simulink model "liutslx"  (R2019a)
settings: configuration reference "configurationSettings" (kept in a data dictionary, not in this file)
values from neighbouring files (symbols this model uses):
  ag = NaN(L.ng,1)    [bdet.m]
  D = meqp()    [fbtp.m]
  dr2FA = dr2Fs(1:nA,1)    [asxycs.m]
  drzFA = drzFs(1:nA,1)    [asxycs.m]
  dz = dzxs(is)    [asxycsJac.m]    (also in bintc.m = (z - zx(kz))/dzx)
  dz2FA = dz2Fs(1:nA,1)    [asxycs.m]
  err = [IaeH            ; IoeH               ; IueH               ; DeH               ; FeH            ; BeH               ; BeH               ; BeH               ; CeH               ; CeH               ; CeH               ; VeH                ; VeH                ; VeH               ]    [fbtopt.m]
  FA = Fs(1:nA,1)    [asxycs.m]    (also in bfhelp.m = [-1                        0        0       ])
  FB = [0                         1        1       ]    [bfhelp.m]
  Fx = meqFx(L,Iy,[Ia;Iu])    [bdet.m]    (also in bfhelp.m = zeros(n+2,3); Fx(2:end-1,2) = FN)
  FX = Fs(nA+1:ns,1)    [asxycs.m]
  Iy = LXt.Iy    [bdet.m]    (also in fbtinit.m = meqinitIy(L,LXs.t,IpD,bbs,LXs.capaj))
  L = fbtc(P,G)    [fbt.m]    (also in fbtc.m = meqc(P,G); fbte.m = varargout{1})
  nA = numel(rA)    [asxycs.m]
  niter = L.P.itercs    [asxycs.m]
  Opy = logical(Opy)    [bfct.m]    (also in bfdoublet.m = Opy==1 | Opy==2)
  rA = rs(1:nA,1)    [asxycs.m]    (also in fbtptcv.m = (rA1 + 3*rA2)/4)
  rX = rs(nA+1:ns,1)    [asxycs.m]    (also in fbtptcv.m = rzbro(iX,1); fbtxana.m = r0)
  zA = zs(1:nA,1)    [asxycs.m]    (also in fbtptcv.m = (zA1 + 3*zA2)/4)
  zX = zs(nA+1:ns,1)    [asxycs.m]    (also in fbtptcv.m = rzbro(iX,2); fbtxana.m = 0)
undefined symbols (not defined in the file or in its folder): Bm, bp, bpli2, Brn, Brrn, Brzn, bt, Bzn, Bzrn, Bzzn, dzg, Ff, Fn, Ft, Ft0, Ie, Ip, iTQ, lB, li, lX, mu, nX, PpQ, PQ, rB, rBt, repmat, Row, rst, TQ, TTpQ, Un, vector, Vp, Wk, WN, Wp, Wt, Wt0, zB
libraries: liulib x34, mkllib x28, simulink x5
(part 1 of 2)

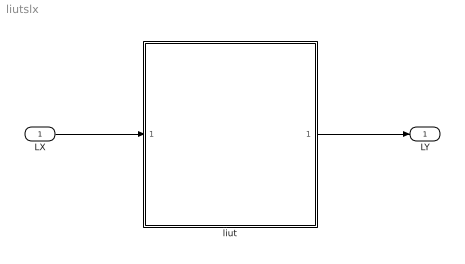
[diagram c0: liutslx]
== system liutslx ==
  LX : Inport  OutDataTypeStr=Bus: LXbus  PortDimensions=1  SampleTime=L.dt  Interpolate=off
  liut : Subsystem  AncestorBlock=liulib/liut  TreatAsAtomicUnit=on
  LY : Outport  OutDataTypeStr=Bus: LYbus  PortDimensions=1
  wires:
  LX/1 -> liut/1(LX)
  liut/1(LY) -> LY/1

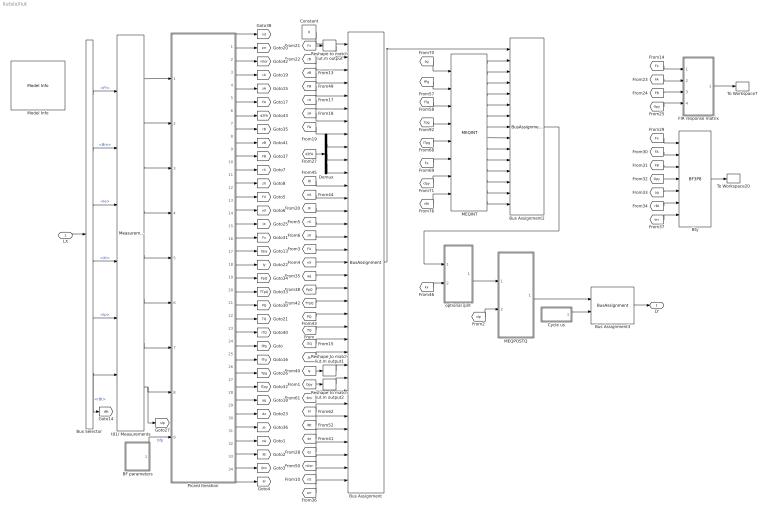
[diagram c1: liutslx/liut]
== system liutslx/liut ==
  LX : Inport
  BF parameters : Subsystem  Variant=on  VariantControl=Variant1
  Bty : liulib/BF3P8  Commented=on  ids=L.idsx  iry=L.iry
  Bus Assignment : BusAssignment  AssignedSignals=Fx,rB,zB,FB,rA,zA,FA,dr2FA,dz2FA,drzFA,lB,nA,lX,rX,zX,FX,nX,ag,PpQ,TTpQ,PQ,TQ,iTQ,Ie,Iy,Opy,Bm,Ff,rBt,dz,dzg,niter,rst,err
  Bus Assignment2 : BusAssignment  AssignedSignals=Ip,Wk,Wp,Wt,Wt0,Ft,Ft0,Vp,bp,bt,mu,li,bpli2,WN
  Bus Assignment3 : BusAssignment  AssignedSignals=cycle
  Bus Selector : BusSelector  OutputSignals=Ff,Bm,Ie,Xt,Ip,rBt
  Constant : Constant  Value=0  OutDataTypeStr=Bus: LYbus
  Cycle us : Subsystem
  Demux : Demux  Outputs=3
  FIR response matrix : Subsystem  Commented=on
  MEQINT : liulib/MEQINT  SystemSampleTime=-1
  MEQPOSTQ : Subsystem  Variant=on  VariantControl=Variant1
  Model Info : simulink/Model-Wide Utilities/Model Info  Frame=on  DisplayStringWithTags=|  HorizontalTextAlignment=Center  LeftAlignmentValue=0.5
      | Model Info
      | %<Creator>
      | %<ModifiedBy>
      | %<ModifiedDate>
      | %<ModifiedComment>
      | %<ModelVersion>
  Picard Iteration : Subsystem
  Reshape to match liut.m output : Reshape  OutputDimensionality=Customize  OutputDimensions=[L.nzx,L.nrx]
  Reshape to match liut.m output1 : Reshape  OutputDimensionality=Customize  OutputDimensions=[L.nzy,L.nry]
  Reshape to match liut.m output2 : Reshape  OutputDimensionality=Customize  OutputDimensions=[L.nzy,L.nry]
  To Workspace20 : ToWorkspace  VariableName=Bty  SampleTime=-1
  To Workspace7 : ToWorkspace  VariableName=Tdg  SampleTime=-1
  optional qint : Subsystem  Variant=on  VariantControl=Variant1
  t01/ Measurements : liulib/t01// Measurements  SystemSampleTime=-1
  LY : Outport
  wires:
  Picard Iteration/13(Out31) -> [FX]
  t01/ Measurements/5 -> Picard Iteration/5(Ip)
  Reshape to match liut.m output2/1 -> Bus Assignment/27
  [Opy] -> Reshape to match liut.m output2/1
  [err] -> Bus Assignment/35
  [rst] -> Bus Assignment/34
  [niter] -> Bus Assignment/33
  [dz] -> Bus Assignment/32
  [dz] -> Bus Assignment/31
  [Ff] -> Bus Assignment/29
  [rBt] -> Bus Assignment/30
  [Bm] -> Bus Assignment/28
  MEQPOSTQ/1(" LYo") -> Bus Assignment3/1
  [sIp] -> MEQPOSTQ/2("sIp ")
  optional qint/1(" LYo") -> MEQPOSTQ/1("LY ")
  t01/ Measurements/1 -> Picard Iteration/1(Yr)
  Bus Selector/2 -> t01/ Measurements/2  "<Bm>"
  Bus Selector/1 -> t01/ Measurements/1  "<Ff>"
  t01/ Measurements/2 -> Picard Iteration/2(Yd)
  t01/ Measurements/3 -> Picard Iteration/3(Yi)
  t01/ Measurements/6 -> Picard Iteration/6(rBt)
  t01/ Measurements/7 -> Picard Iteration/7(FN)
  t01/ Measurements/8 -> [sIp], Picard Iteration/8(sIp)
  BF parameters/1(" bfp") -> Picard Iteration/9(bfp)  "bfp"
  LX/1 -> Bus Selector/1
  Bus Selector/5 -> t01/ Measurements/5  "<Ip>"
  Bus Selector/3 -> t01/ Measurements/3  "<Ie>"
  t01/ Measurements/4 -> Picard Iteration/4(Ie)
  MEQINT/5 -> Bus Assignment2/6
  [ag] -> MEQINT/1
  [Opy] -> MEQINT/7
  [fTg] -> MEQINT/3
  MEQINT/3 -> Bus Assignment2/4
  [fPg] -> MEQINT/2
  MEQINT/6 -> Bus Assignment2/7
  [rBt] -> MEQINT/8
  MEQINT/9 -> Bus Assignment2/10
  MEQINT/7 -> Bus Assignment2/8
  MEQINT/12 -> Bus Assignment2/13
  MEQINT/1 -> Bus Assignment2/2
  [Fx] -> MEQINT/6
  MEQINT/2 -> Bus Assignment2/3
  [Tpg] -> MEQINT/4
  MEQINT/4 -> Bus Assignment2/5
  [ITpg] -> MEQINT/5
  MEQINT/8 -> Bus Assignment2/9
  MEQINT/11 -> Bus Assignment2/12
  MEQINT/10 -> Bus Assignment2/11
  Constant/1 -> Bus Assignment/1
  Picard Iteration/8(Out9) -> [rB]
  Picard Iteration/6(Out7) -> [FA]
  Picard Iteration/24(Out19) -> [fPg]
  Picard Iteration/9(Out10) -> [zB]
  Picard Iteration/4(Out5) -> [rA]
  Picard Iteration/2(Out2) -> [err]
  Picard Iteration/21(Out16) -> [PQ]
  Picard Iteration/7(Out8) -> [d2FA]
  Picard Iteration/25(Out20) -> [fTg]
  Picard Iteration/26(Out21) -> [Tpg]
  Picard Iteration/28(Out23) -> [ag]
  Picard Iteration/16(Out13) -> [Fx]
  Picard Iteration/3(Out3) -> [niter]
  Picard Iteration/1(Out1) -> [rst]
  Picard Iteration/15(Out12) -> [lX]
  Picard Iteration/17(Out14) -> [Opy]
  Picard Iteration/22(Out17) -> [TQ]
  Picard Iteration/27(Out22) -> [ITpg]
  Picard Iteration/10(Out11) -> [FB]
  Picard Iteration/20(Out26) -> [TTpQ]
  Picard Iteration/30(Out4) -> [Je]
  Picard Iteration/5(Out6) -> [zA]
  Picard Iteration/18(Out15) -> [Iy]
  Picard Iteration/29(Out24) -> [dz]
  Picard Iteration/19(Out25) -> [PpQ]
  Picard Iteration/23(Out18) -> [iTQ]
  [rA] -> Bus Assignment/6
  [zA] -> Bus Assignment/7
  [FA] -> Bus Assignment/8
  Demux/1 -> Bus Assignment/9
  Demux/3 -> Bus Assignment/11
  Demux/2 -> Bus Assignment/10
  [d2FA] -> Demux/1
  [FB] -> Bus Assignment/5
  [zB] -> Bus Assignment/4
  [rB] -> Bus Assignment/3
  [Fx] -> Reshape to match liut.m output/1
  Picard Iteration/31(Out27) -> [nA]
  Picard Iteration/32(Out28) -> [lB]
  [lB] -> Bus Assignment/12
  [nA] -> Bus Assignment/13
  [ag] -> Bus Assignment/19
  [lX] -> Bus Assignment/14
  [PpQ] -> Bus Assignment/20
  [TTpQ] -> Bus Assignment/21
  [PQ] -> Bus Assignment/22
  [TQ] -> Bus Assignment/23
  Bus Assignment/1 -> Bus Assignment2/1
  MEQINT/13 -> Bus Assignment2/14
  Reshape to match liut.m output/1 -> Bus Assignment/2
  Cycle us/1(Out1) -> Bus Assignment3/2
  Bus Assignment3/1 -> LY/1
  [err] -> Bty/7
  [FB] -> Bty/3
  [Fx] -> Bty/1
  [FB] -> FIR response matrix/3(FB)
  [ag] -> Bty/5
  [Fx] -> FIR response matrix/1(Fx)
  Bty/1 -> To Workspace20/1
  [rBt] -> Bty/6
  [Opy] -> Bty/4
  FIR response matrix/1(Tdg) -> To Workspace7/1
  [FA] -> FIR response matrix/2(FA)
  [FA] -> Bty/2
  [Opy] -> FIR response matrix/4(Opy)
  Bus Selector/4 -> t01/ Measurements/4  "<Xt>"
  Bus Selector/6 -> [rBt], t01/ Measurements/6  "<rBt>"
  [Je] -> Bus Assignment/25
  [Iy] -> Reshape to match liut.m output1/1
  Reshape to match liut.m output1/1 -> Bus Assignment/26
  [iTQ] -> Bus Assignment/24
  MEQINT/14 -> Bus Assignment2/15
  Picard Iteration/33(Out29) -> [Bm]
  Picard Iteration/34(Out30) -> [Ff]
  [Fx] -> optional qint/2(Fx)
  Bus Assignment2/1 -> optional qint/1("LY ")
  [FX] -> Bus Assignment/17
  Picard Iteration/14(Out32) -> [nX]
  [nX] -> Bus Assignment/18
  Picard Iteration/11(Out33) -> [rX]
  Picard Iteration/12(Out34) -> [zX]
  [rX] -> Bus Assignment/15
  [zX] -> Bus Assignment/16

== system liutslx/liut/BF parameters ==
  BF3I : Subsystem  VariantControl=liuBFCTMODEvariant2
  BF3P : Subsystem  VariantControl=liuBFCTMODEvariant1
  BFEF : Subsystem  VariantControl=liuBFCTMODEvariant3
  " bfp" : Outport

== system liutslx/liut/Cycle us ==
  Data Type Conversion : DataTypeConversion
  Memory : Memory  InheritSampleTime=on
  Sum : Sum  Inputs=|+-
  Wall time : liulib/Wall time  f=1000000
  Out1 : Outport  OutDataTypeStr=single
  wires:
  Wall time/1 -> Sum/1, Memory/1
  Sum/1 -> Data Type Conversion/1
  Memory/1 -> Wall time/1, Sum/2
  Data Type Conversion/1 -> Out1/1

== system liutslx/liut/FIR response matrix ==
  Fx : Inport
  FA : Inport  Port=2
  FB : Inport  Port=3
  Opy : Inport  Port=4
  BF3I4 : liulib/BF3I4  nzy=L.nzy  nry=L.nry
  Constant : Constant  Value=ones(21,3)  VectorParams1D=off  OutDataTypeStr=single
  Constant1 : Constant  Value=0:9  OutDataTypeStr=uint32
  Constant2 : Constant  Value=[ones(10,1) zeros(10,1)]  OutDataTypeStr=single
  Terminator : Terminator
  Tdg : Outport
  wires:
  BF3I4/2 -> Terminator/1
  Fx/1 -> BF3I4/1
  Opy/1 -> BF3I4/4
  Constant2/1 -> BF3I4/7
  FA/1 -> BF3I4/2
  Constant1/1 -> BF3I4/6
  Constant/1 -> BF3I4/5
  BF3I4/1 -> Tdg/1
  FB/1 -> BF3I4/3

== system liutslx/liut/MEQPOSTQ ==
  "LY " : Inport
  "sIp " : Inport  Port=2
  Direct pass : Subsystem  VariantControl=liuITERQMODEvariant0
  MEQPOSTQ : liulib/MEQPOSTQ  SystemSampleTime=-1  VariantControl=liuITERQMODEvariant1
  " LYo" : Outport

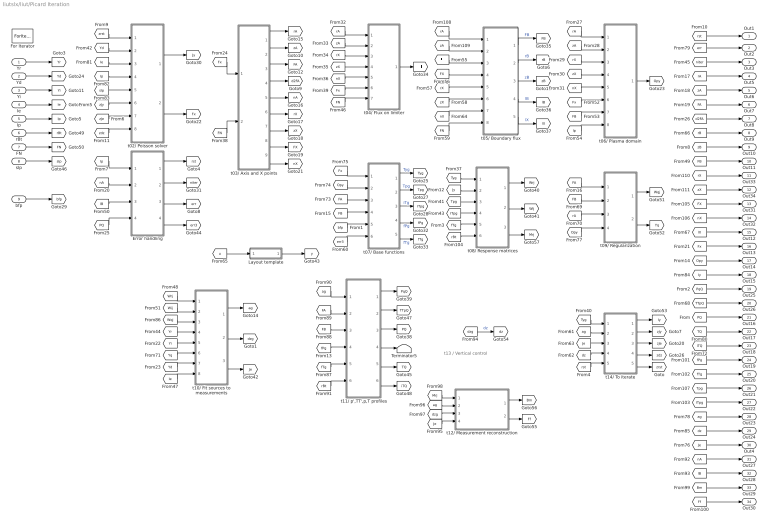
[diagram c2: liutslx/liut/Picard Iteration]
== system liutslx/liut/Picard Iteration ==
  note: t13 / Vertical control
  Yr : Inport
  Yd : Inport  Port=2
  Yi : Inport  Port=3
  Ie : Inport  Port=4
  Ip : Inport  Port=5
  rBt : Inport  Port=6
  FN : Inport  Port=7
  sIp : Inport  Port=8
  bfp : Inport  Port=9
  Error handling : Subsystem
  For Iterator : ForIterator  IterationLimit=L.P.itert  ShowIterationPort=off
  Layout template : Subsystem  Commented=on
  Terminator5 : Terminator
  t02/ Poisson solver : Subsystem
  t03/ Axis and X points : Subsystem  TreatAsAtomicUnit=on
  t04/ Flux on limiter : Subsystem
  t05/ Boundary flux : Subsystem
  t06/ Plasma domain : Subsystem
  t07/ Base functions : Subsystem  Variant=on
  t08/ Response matrices : Subsystem
  t09/ Regularization : Subsystem  TreatAsAtomicUnit=on
  t10/ Fit sources to measurements : Subsystem  Variant=on  VariantControl=Variant1
  t11/ p',TT',p,T profiles : Subsystem  VariantControl=Variant1
  t12/ Measurement reconstruction : Subsystem
  t14/ To iterate : Subsystem
  Out1 : Outport
  Out2 : Outport  Port=2
  Out3 : Outport  Port=3
  Out5 : Outport  Port=4
  Out6 : Outport  Port=5
  Out7 : Outport  Port=6
  Out8 : Outport  Port=7
  Out9 : Outport  Port=8
  Out10 : Outport  Port=9
  Out11 : Outport  Port=10
  Out33 : Outport  Port=11
  Out34 : Outport  Port=12
  Out31 : Outport  Port=13
  Out32 : Outport  Port=14
  Out12 : Outport  Port=15
  Out13 : Outport  Port=16
  Out14 : Outport  Port=17
  Out15 : Outport  Port=18
  Out25 : Outport  Port=19
  Out26 : Outport  Port=20
  Out16 : Outport  Port=21
  Out17 : Outport  Port=22
  Out18 : Outport  Port=23
  Out19 : Outport  Port=24
  Out20 : Outport  Port=25
  Out21 : Outport  Port=26
  Out22 : Outport  Port=27
  Out23 : Outport  Port=28
  Out24 : Outport  Port=29
  Out4 : Outport  Port=30
  Out27 : Outport  Port=31
  Out28 : Outport  Port=32
  Out29 : Outport  Port=33
  Out30 : Outport  Port=34
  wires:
  [rA] -> t05/ Boundary flux/1(rA)
  [zA] -> t05/ Boundary flux/2(zA)
  t05/ Boundary flux/5(lX) -> [lX]  "lX"
  t05/ Boundary flux/1(FB) -> [FB]  "FB"
  t05/ Boundary flux/4(lB) -> [lB]  "lB"
  t05/ Boundary flux/3(zB) -> [zB]  "zB"
  t05/ Boundary flux/2(rB) -> [rB]  "rB"
  [FN] -> t05/ Boundary flux/8(FN)
  [zX] -> t05/ Boundary flux/6(zX)
  [rX] -> t05/ Boundary flux/5(rX)
  [Fl] -> t05/ Boundary flux/3(Fl)
  [FX] -> t05/ Boundary flux/4(FX)
  [nX] -> t05/ Boundary flux/7(nX)
  [FX] -> Out31/1
  [rBt] -> t08/ Response matrices/6(rBt)
  [Je] -> Out4/1
  [Wqj] -> t10/ Fit sources to measurements/3(Wqj)
  [Yq] -> t10/ Fit sources to measurements/6(Yq)
  [FA] -> t09/ Regularization/1(FA)
  [FB] -> t09/ Regularization/2(FB)
  [Opy] -> t09/ Regularization/4(Opy)
  [rA] -> t09/ Regularization/3(rA)
  t09/ Regularization/2(Yq) -> [Yq]
  t09/ Regularization/1(Wqj) -> [Wqj]
  t10/ Fit sources to measurements/3(Je) -> [Je]
  t10/ Fit sources to measurements/2(dzg) -> [dzg]
  t10/ Fit sources to measurements/1(ag) -> [ag]
  [Ie] -> t10/ Fit sources to measurements/8(Ie)
  [Yd] -> t10/ Fit sources to measurements/7(Yd)
  [Yi] -> t10/ Fit sources to measurements/5(Yi)
  [Yr] -> t10/ Fit sources to measurements/4(Yr)
  [Wij] -> t10/ Fit sources to measurements/2(Wij)
  [Wrj] -> t10/ Fit sources to measurements/1(Wrj)
  Error handling/4(err3) -> [err3]
  t07/ Base functions/3(ITpg) -> [ITpg]  "iTg"
  t07/ Base functions/2(Tpg) -> [Tpg]  "Tpg"
  [zA] -> t04/ Flux on limiter/2(zA)
  [rA] -> t04/ Flux on limiter/1(rA)
  [u] -> Layout template/1(u)
  Layout template/1(y) -> [y]
  [PQ] -> Out16/1
  [Iy] -> Out15/1
  [PQ] -> Error handling/4(PQ)
  [nA] -> Error handling/2(nA)
  [Ip] -> Error handling/1(Ip)
  [Fx] -> Out13/1
  [FB] -> Out11/1
  [Opy] -> Out14/1
  t11/ p',TT',p,T profiles/3(PQ) -> [PQ]
  [lX] -> Out12/1
  [rB] -> Out9/1
  [rA] -> Out5/1
  [zA] -> Out6/1
  t04/ Flux on limiter/1(Fl) -> [Fl]
  [ITpg] -> t08/ Response matrices/4(ITpg)
  [fPg] -> Out19/1
  [fTg] -> Out20/1
  [Tpg] -> Out21/1
  [nX] -> t04/ Flux on limiter/5(nX)
  [rX] -> t04/ Flux on limiter/3(rX)
  [zX] -> t04/ Flux on limiter/4(zX)
  [rX] -> t06/ Plasma domain/3(rX)
  [rA] -> t06/ Plasma domain/1(rA)
  [fTg] -> t11/ p',TT',p,T profiles/5(fTg)
  [FB] -> t11/ p',TT',p,T profiles/3(FB)
  [zrst] -> t02/ Poisson solver/1(rst)
  Ie/1 -> [Ie]
  Yd/1 -> [Yd]
  [Fx] -> t04/ Flux on limiter/6(Fx)
  [FN] -> t04/ Flux on limiter/7(FN)
  bfp/1 -> [bfp]
  Ip/1 -> [Ip]
  Yi/1 -> [Yi]
  Yr/1 -> [Yr]
  [zJe] -> t02/ Poisson solver/7(zJe)
  [Yd] -> t02/ Poisson solver/2(Yd)
  [zJy] -> t02/ Poisson solver/6(zJy)
  [iTQ] -> Out18/1
  t11/ p',TT',p,T profiles/6(iTQ) -> [iTQ]
  t11/ p',TT',p,T profiles/5(TQ) -> [TQ]
  [nX] -> t06/ Plasma domain/5(nX)
  [zX] -> t06/ Plasma domain/4(zX)
  [zA] -> t06/ Plasma domain/2(zA)
  t08/ Response matrices/2(Wij) -> [Wij]
  [fTg] -> t08/ Response matrices/5(fTg)
  t11/ p',TT',p,T profiles/4(hqTQ) -> Terminator5/1
  t11/ p',TT',p,T profiles/2(TTpQ) -> [TTpQ]
  t11/ p',TT',p,T profiles/1(PpQ) -> [PqQ]
  [Tpg] -> t08/ Response matrices/3(Tpg)
  [Tyg] -> t08/ Response matrices/1(Tyg)
  t06/ Plasma domain/1(Opy) -> [Opy]
  [Jy] -> t08/ Response matrices/2(Jy)
  [rst] -> Out1/1
  [sIp] -> t02/ Poisson solver/5(sIp)
  sIp/1 -> [sIp]
  t07/ Base functions/5(fTg) -> [fTg]  "fTg"
  t07/ Base functions/4(fPg) -> [fPg]  "fPg"
  [bfp] -> t07/ Base functions/5(bfp)
  t07/ Base functions/1(Tyg) -> [Tyg]  "Tyg"
  [err3] -> t07/ Base functions/6(err)
  [FB] -> t07/ Base functions/4(FB)
  [FA] -> Out7/1
  [d2FA] -> Out8/1
  [ag] -> Out23/1
  [err] -> Out2/1
  [rBt] -> t11/ p',TT',p,T profiles/6(rBt)
  [Ip] -> t02/ Poisson solver/4(Ip)
  [Ie] -> t02/ Poisson solver/3(Ie)
  [TQ] -> Out17/1
  [Ip] -> t06/ Plasma domain/8(Ip)
  [FB] -> t06/ Plasma domain/7(FB)
  [Fx] -> t06/ Plasma domain/6(Fx)
  Error handling/3(err) -> [err]
  [lB] -> Error handling/3(lB)
  [niter] -> Out3/1
  [dz] -> Out24/1
  t02/ Poisson solver/2(Fx) -> [Fx]
  [zdz] -> t02/ Poisson solver/8(zdz)
  t02/ Poisson solver/1(Jy) -> [Jy]
  [FA] -> t07/ Base functions/3(FA)
  [Opy] -> t07/ Base functions/2(Opy)
  [Fx] -> t07/ Base functions/1(Fx)
  t08/ Response matrices/1(Wrj) -> [Wrj]
  Error handling/1(rst) -> [rst]
  Error handling/2(niter) -> [niter]
  [zB] -> Out10/1
  FN/1 -> [FN]
  rBt/1 -> [rBt]
  [ITpg] -> Out22/1
  [FA] -> t11/ p',TT',p,T profiles/2(FA)
  [ag] -> t11/ p',TT',p,T profiles/1(ag)
  [fPg] -> t11/ p',TT',p,T profiles/4(fPg)
  [rst] -> t14/ To iterate/5(rst)
  [ag] -> t14/ To iterate/2(ag)
  [Tyg] -> t14/ To iterate/1(Tyg)
  [Je] -> t14/ To iterate/3(Je)
  [dz] -> t14/ To iterate/4(dz)
  t14/ To iterate/2(zJy) -> [zJy]
  t14/ To iterate/3(zJe) -> [zJe]
  t14/ To iterate/4(zdz) -> [zdz]
  t14/ To iterate/5(zrst) -> [zrst]
  [PqQ] -> Out25/1
  [TTpQ] -> Out26/1
  t14/ To iterate/1(Iy) -> [Iy]
  [nA] -> Out27/1
  [lB] -> Out28/1
  [dzg] -> [dz]  "dz"
  t12/ Measurement reconstruction/1(Bm) -> [Bm]
  t12/ Measurement reconstruction/2(Ff) -> [Ff]
  [Mrj] -> t12/ Measurement reconstruction/1(Mrj)
  [ag] -> t12/ Measurement reconstruction/2(ag)
  [dzg] -> t12/ Measurement reconstruction/3(dzg)
  t08/ Response matrices/3(Mrj) -> [Mrj]
  [Je] -> t12/ Measurement reconstruction/4(Ie)
  [Ff] -> Out30/1
  [Bm] -> Out29/1
  [nX] -> Out32/1
  [rX] -> Out33/1
  [zX] -> Out34/1
  [Fx] -> t03/ Axis and X points/1(Fx)
  [FN] -> t03/ Axis and X points/2(FN)
  t03/ Axis and X points/1(rA) -> [rA]
  t03/ Axis and X points/2(zA) -> [zA]
  t03/ Axis and X points/3(FA) -> [FA]
  t03/ Axis and X points/4(d2FA) -> [d2FA]
  t03/ Axis and X points/5(nA) -> [nA]
  t03/ Axis and X points/6(rX) -> [rX]
  t03/ Axis and X points/7(zX) -> [zX]
  t03/ Axis and X points/8(FX) -> [FX]
  t03/ Axis and X points/9(nX) -> [nX]

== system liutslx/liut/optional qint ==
  "LY " : Inport
  Fx : Inport  Port=2
  direct pass : Subsystem  VariantControl=liuINFCTMODEvariant1
  "qint " : Subsystem  VariantControl=liuINFCTMODEvariant2
  " LYo" : Outport

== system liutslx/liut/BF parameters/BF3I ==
  BF3I parameters : Subsystem
  Bus Creator : BusCreator  Inputs=4
  bfp : Outport
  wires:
  BF3I parameters/1(gNg) -> Bus Creator/1
  Bus Creator/1 -> bfp/1
  BF3I parameters/3(fPg) -> Bus Creator/3
  BF3I parameters/4(fTg) -> Bus Creator/4
  BF3I parameters/2(IgNg) -> Bus Creator/2

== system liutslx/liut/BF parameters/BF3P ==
  Constant : Constant  Value=L.P.bfp
  bfp : Outport
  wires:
  Constant/1 -> bfp/1

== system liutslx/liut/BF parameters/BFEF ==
  Constant : Constant  Value=L.P.bfp
  bfp : Outport
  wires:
  Constant/1 -> bfp/1

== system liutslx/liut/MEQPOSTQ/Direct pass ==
  "LY " : Inport
  "sIp " : Inport  Port=2
  Terminator : Terminator
  " LYo" : Outport
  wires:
  "sIp "/1 -> Terminator/1
  "LY "/1 -> " LYo"/1

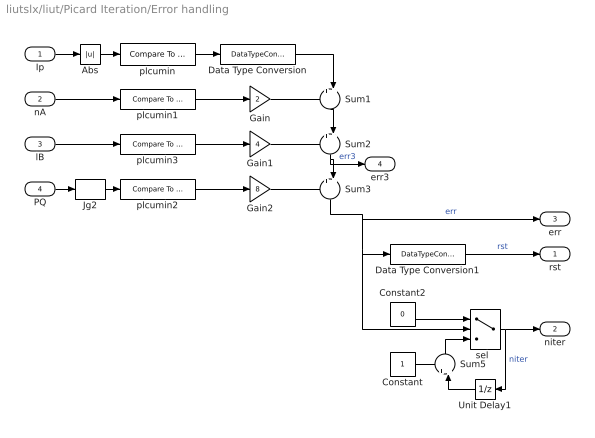
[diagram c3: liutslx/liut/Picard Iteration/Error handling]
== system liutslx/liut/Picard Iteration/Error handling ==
  Ip : Inport
  nA : Inport  Port=2
  lB : Inport  Port=3
  PQ : Inport  Port=4
  Abs : Abs
  Constant : Constant  VectorParams1D=off  OutDataTypeStr=int32
  Constant2 : Constant  Value=0  VectorParams1D=off  OutDataTypeStr=int32
  Data Type Conversion : DataTypeConversion  OutDataTypeStr=int32
  Data Type Conversion1 : DataTypeConversion  OutDataTypeStr=boolean
  Gain : Gain  Gain=2  OutDataTypeStr=int32
  Gain1 : Gain  Gain=4  OutDataTypeStr=int32
  Gain2 : Gain  Gain=8  OutDataTypeStr=int32
  Jg2 : Selector  IndexMode=Zero-based  IndexOptions=Index vector (dialog)  Indices=0  OutputSizes=1
  Sum{1..3,5} (4 alike) : Sum  Inputs=++|
  Unit Delay1 : UnitDelay  InitialCondition=int32(0)  SampleTime=-1  HasFrameUpgradeWarning=on
  plcumin : simulink/Logic and Bit Operations/Compare To Constant  relop=<  const=L.P.Ipmin  OutDataTypeStr=uint8
  plcumin1 : simulink/Logic and Bit Operations/Compare To Constant  relop===  const=0  OutDataTypeStr=uint8
  plcumin2 : simulink/Logic and Bit Operations/Compare To Constant  relop=<  const=0  OutDataTypeStr=uint8
  plcumin3 : simulink/Logic and Bit Operations/Compare To Constant  relop===  const=0  OutDataTypeStr=uint8
  "sel  " : Switch  Criteria=u2 ~= 0  OutDataTypeStr=int32
  rst : Outport
  niter : Outport  Port=2
  err : Outport  Port=3
  err3 : Outport  Port=4
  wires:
  Sum2/1 -> Sum3/2, err3/1  "err3"
  Sum1/1 -> Sum2/2
  Data Type Conversion/1 -> Sum1/2
  Gain/1 -> Sum1/1
  Sum3/1 -> err/1, Data Type Conversion1/1, "sel  "/2  "err"
  Gain2/1 -> Sum3/1
  Gain1/1 -> Sum2/1
  plcumin/1 -> Data Type Conversion/1
  plcumin1/1 -> Gain/1
  Constant2/1 -> "sel  "/1
  Unit Delay1/1 -> Sum5/2
  plcumin3/1 -> Gain1/1
  lB/1 -> plcumin3/1
  Constant/1 -> Sum5/1
  Sum5/1 -> "sel  "/3
  "sel  "/1 -> Unit Delay1/1, niter/1  "niter"
  Abs/1 -> plcumin/1
  Ip/1 -> Abs/1
  Data Type Conversion1/1 -> rst/1  "rst"
  PQ/1 -> Jg2/1
  Jg2/1 -> plcumin2/1
  nA/1 -> plcumin1/1
  plcumin2/1 -> Gain2/1

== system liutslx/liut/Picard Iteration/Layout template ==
  u : Inport
  y : Outport
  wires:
  u/1 -> y/1

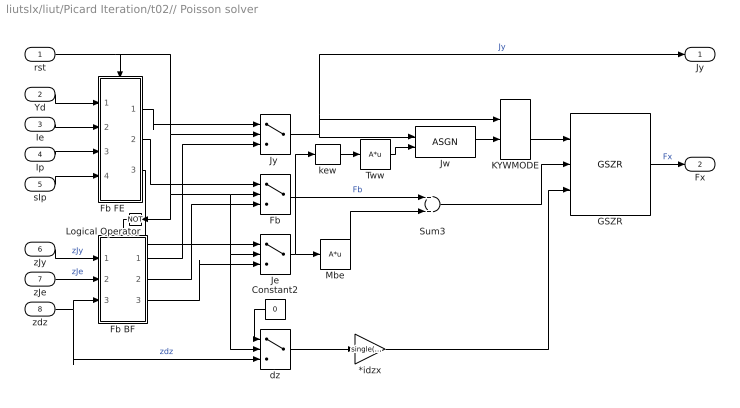
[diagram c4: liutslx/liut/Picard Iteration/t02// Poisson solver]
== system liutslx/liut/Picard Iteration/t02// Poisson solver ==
  rst : Inport
  Yd : Inport  Port=2
  Ie : Inport  Port=3
  Ip : Inport  Port=4
  sIp : Inport  Port=5
  zJy : Inport  Port=6
  zJe : Inport  Port=7
  zdz : Inport  Port=8
  *idzx : Gain  Gain=single(L.idzx)
  Constant2 : Constant  Value=0  OutDataTypeStr=single
  Fb : Switch  Criteria=u2 ~= 0
  Fb BF : Subsystem  TreatAsAtomicUnit=on
  Fb FE : Subsystem  TreatAsAtomicUnit=on
  GSZR : liulib/GSZR  cx=L.cx  cq=L.cq  cr=L.cr  cs=L.cs  ci=L.ci  co=L.co
  Je : Switch  Criteria=u2 ~= 0
  Jw : liulib/ASGN  iu=L.kyw-1
  "Jy " : Switch  Criteria=u2 ~= 0
  KYWMODE : VariantSource
  Logical Operator : Logic  Operator=NOT  IconShape=distinctive  AllPortsSameDT=off  OutDataTypeStr=boolean
  Mbe : mkllib/A*u  A=L.Mbe
  Sum3 : Sum
  Tww : mkllib/A*u  A=single(L.Tww)
  dz : Switch  Criteria=u2 ~= 0
  kew : Selector  IndexMode=Zero-based  IndexOptions=Index vector (dialog)  Indices=L.kew-1  OutputSizes=1
  Jy : Outport
  Fx : Outport  Port=2
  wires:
  *idzx/1 -> GSZR/3
  Sum3/1 -> GSZR/2
  KYWMODE/1 -> GSZR/1
  Jw/1 -> KYWMODE/2
  Fb BF/1(=Jy) -> "Jy "/3
  Fb BF/3(=Je) -> Je/3
  sIp/1 -> Fb FE/4(sIp)
  Ip/1 -> Fb FE/3(Ip)
  Ie/1 -> Fb FE/2(Ie)
  Constant2/1 -> dz/1
  dz/1 -> *idzx/1
  Fb FE/1(Jy) -> "Jy "/1
  Tww/1 -> Jw/2
  Fb BF/2(Fb) -> Fb/3
  Fb FE/2(Fb) -> Fb/1
  Fb FE/3(Je) -> Je/1
  "Jy "/1 -> Jy/1, KYWMODE/1, Jw/1  "Jy"
  Fb/1 -> Sum3/1  "Fb"
  Je/1 -> kew/1, Mbe/1
  Mbe/1 -> Sum3/2
  zJy/1 -> Fb BF/1(Jy)  "zJy"
  Logical Operator/1 -> Fb BF/Enable
  rst/1 -> "Jy "/2, Logical Operator/1, dz/2, Je/2, Fb/2, Fb FE/Enable
  kew/1 -> Tww/1
  zJe/1 -> Fb BF/2(Je)  "zJe"
  zdz/1 -> Fb BF/3(dz), dz/3  "zdz"
  GSZR/1 -> Fx/1  "Fx"
  Yd/1 -> Fb FE/1(Yd)

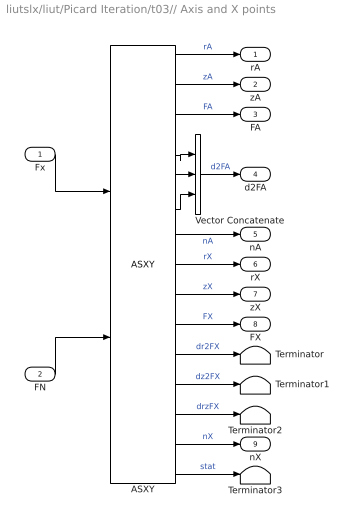
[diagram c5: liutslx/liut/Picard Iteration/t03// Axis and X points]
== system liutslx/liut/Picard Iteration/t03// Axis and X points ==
  Fx : Inport
  FN : Inport  Port=2
  ASXY : liulib/ASXY  rx=L.G.rx  zx=L.G.zx  dr=L.drx  dz=L.dzx  idr=L.idrx  idz=L.idzx  Oasx=L.Oasx  daxm=L.P.dasm
  Terminator{,1..3} (4 alike) : Terminator
  Vector Concatenate : Concatenate  NumInputs=3
  rA : Outport
  zA : Outport  Port=2
  FA : Outport  Port=3
  d2FA : Outport  Port=4
  nA : Outport  Port=5
  rX : Outport  Port=6
  zX : Outport  Port=7
  FX : Outport  Port=8
  nX : Outport  Port=9
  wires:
  Vector Concatenate/1 -> d2FA/1  "d2FA"
  ASXY/7 -> nA/1  "nA"
  ASXY/12 -> Terminator1/1  "dz2FX"
  ASXY/2 -> zA/1  "zA"
  ASXY/14 -> nX/1  "nX"
  FN/1 -> ASXY/2
  ASXY/13 -> Terminator2/1  "drzFX"
  ASXY/3 -> FA/1  "FA"
  ASXY/11 -> Terminator/1  "dr2FX"
  ASXY/15 -> Terminator3/1  "stat"
  ASXY/6 -> Vector Concatenate/3
  ASXY/1 -> rA/1  "rA"
  Fx/1 -> ASXY/1
  ASXY/4 -> Vector Concatenate/1
  ASXY/9 -> zX/1  "zX"
  ASXY/10 -> FX/1  "FX"
  ASXY/5 -> Vector Concatenate/2
  ASXY/8 -> rX/1  "rX"

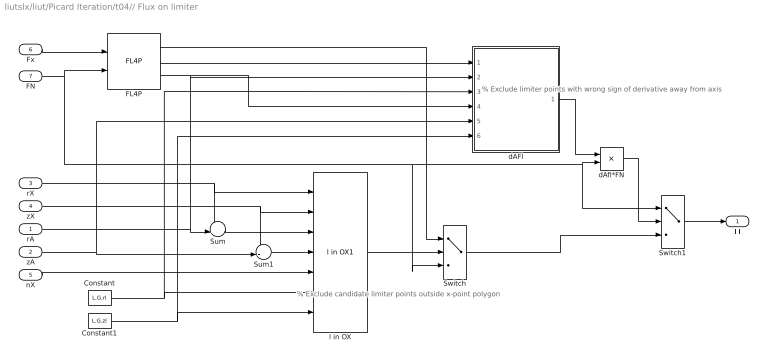
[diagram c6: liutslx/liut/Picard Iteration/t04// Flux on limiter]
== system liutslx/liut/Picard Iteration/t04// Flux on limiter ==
  note: % Exclude candidate limiter points outside x-point polygon
  note: % Exclude limiter points with wrong sign of derivative away from axis
  rA : Inport
  zA : Inport  Port=2
  rX : Inport  Port=3
  zX : Inport  Port=4
  nX : Inport  Port=5
  Fx : Inport  Port=6
  FN : Inport  Port=7
  Constant : Constant  Value=L.G.rl  OutDataTypeStr=single
  Constant1 : Constant  Value=L.G.zl  OutDataTypeStr=single
  FL4P : liulib/FL4P  kl=int32(L.kxl-1)  cl=L.clx  nz=L.nzx
  Sum : Sum  Inputs=-+|
  Sum1 : Sum  Inputs=-+|
  Switch : Switch  Criteria=u2 ~= 0
  Switch1 : Switch  Criteria=u2 > Threshold  ZeroCross=off
  dAFl : Subsystem
  dAfl*FN : Product
  l in OX : liulib/l in OX1  a=0
  Fl : Outport
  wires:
  FL4P/3 -> dAFl/4(dzFl)
  FL4P/2 -> dAFl/1(drFl)
  FN/1 -> FL4P/2, dAfl*FN/2, Switch1/1, Switch/3
  Switch/1 -> Switch1/3
  dAfl*FN/1 -> Switch1/2
  dAFl/1(dAFl) -> dAfl*FN/1
  Switch1/1 -> Fl/1
  Constant1/1 -> dAFl/6(zl), l in OX/7
  Constant/1 -> dAFl/3(rl), l in OX/6
  Fx/1 -> FL4P/1
  Sum1/1 -> l in OX/4
  zA/1 -> Sum1/2, dAFl/5(zA)
  Sum/1 -> l in OX/3
  rA/1 -> Sum/2, dAFl/2(rA)
  zX/1 -> l in OX/2, Sum1/1
  rX/1 -> l in OX/1, Sum/1
  FL4P/1 -> Switch/1
  l in OX/1 -> Switch/2
  nX/1 -> l in OX/5

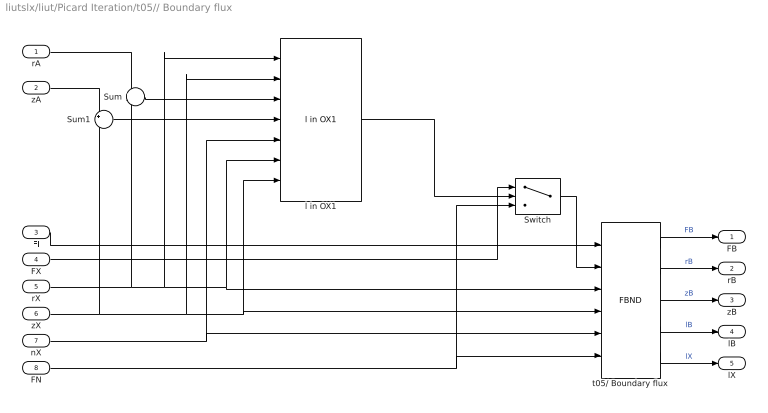
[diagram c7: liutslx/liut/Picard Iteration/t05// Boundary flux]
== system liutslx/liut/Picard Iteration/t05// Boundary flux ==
  rA : Inport
  zA : Inport  Port=2
  Fl : Inport  Port=3
  FX : Inport  Port=4
  rX : Inport  Port=5
  zX : Inport  Port=6
  nX : Inport  Port=7
  FN : Inport  Port=8
  Sum : Sum  Inputs=+-
  Sum1 : Sum  Inputs=+-
  Switch : Switch  Criteria=u2 ~= 0
  l in OX1 : liulib/l in OX1  a=0
  t05/ Boundary flux : liulib/FBND  rl=L.G.rl  zl=L.G.zl
  FB : Outport
  rB : Outport  Port=2
  zB : Outport  Port=3
  lB : Outport  Port=4
  lX : Outport  Port=5
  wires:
  Switch/1 -> t05/ Boundary flux/2
  l in OX1/1 -> Switch/2
  Sum1/1 -> l in OX1/4
  zA/1 -> Sum1/1
  Sum/1 -> l in OX1/3
  rA/1 -> Sum/1
  FN/1 -> t05/ Boundary flux/6, Switch/3
  nX/1 -> t05/ Boundary flux/5, l in OX1/5
  zX/1 -> Sum1/2, t05/ Boundary flux/4, l in OX1/7, l in OX1/2
  rX/1 -> t05/ Boundary flux/3, l in OX1/6, l in OX1/1, Sum/2
  FX/1 -> Switch/1
  t05/ Boundary flux/5 -> lX/1  "lX"
  t05/ Boundary flux/4 -> lB/1  "lB"
  t05/ Boundary flux/3 -> zB/1  "zB"
  t05/ Boundary flux/2 -> rB/1  "rB"
  t05/ Boundary flux/1 -> FB/1  "FB"
  Fl/1 -> t05/ Boundary flux/1

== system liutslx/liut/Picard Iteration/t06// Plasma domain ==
  rA : Inport
  zA : Inport  Port=2
  rX : Inport  Port=3
  zX : Inport  Port=4
  nX : Inport  Port=5
  Fx : Inport  Port=6
  FB : Inport  Port=7
  Ip : Inport  Port=8
  Constant : Constant  Value=L.ry  OutDataTypeStr=Inherit: Inherit via back propagation
  Constant1 : Constant  Value=L.zy  OutDataTypeStr=Inherit: Inherit via back propagation
  Data Type Conversion : DataTypeConversion  OutDataTypeStr=int8
  OXy : liulib/BAVX2  a=0
  PDOM : liulib/PDOM
  Sum : Sum  Inputs=-+|
  Sum1 : Sum  Inputs=-+|
  Opy : Outport
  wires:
  Data Type Conversion/1 -> Opy/1
  PDOM/1 -> Data Type Conversion/1  "Opy"
  zA/1 -> Sum1/2
  Sum1/1 -> OXy/4
  Sum/1 -> OXy/3
  rA/1 -> Sum/2
  zX/1 -> OXy/2, Sum1/1
  rX/1 -> OXy/1, Sum/1
  Constant/1 -> OXy/6
  Constant1/1 -> OXy/7
  OXy/1 -> PDOM/4
  nX/1 -> OXy/5
  Ip/1 -> PDOM/3
  FB/1 -> PDOM/2
  Fx/1 -> PDOM/1

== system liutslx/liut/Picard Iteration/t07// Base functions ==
  Fx : Inport
  Opy : Inport  Port=2
  FA : Inport  Port=3
  FB : Inport  Port=4
  bfp : Inport  Port=5
  err : Inport  Port=6
  bf3i : Subsystem  VariantControl=liuBFCTMODEvariant2
  bf3p : Subsystem  VariantControl=liuBFCTMODEvariant1
  bfef : Subsystem  VariantControl=liuBFCTMODEvariant3
  Tyg : Outport
  Tpg : Outport  Port=2
  ITpg : Outport  Port=3
  fPg : Outport  Port=4
  fTg : Outport  Port=5

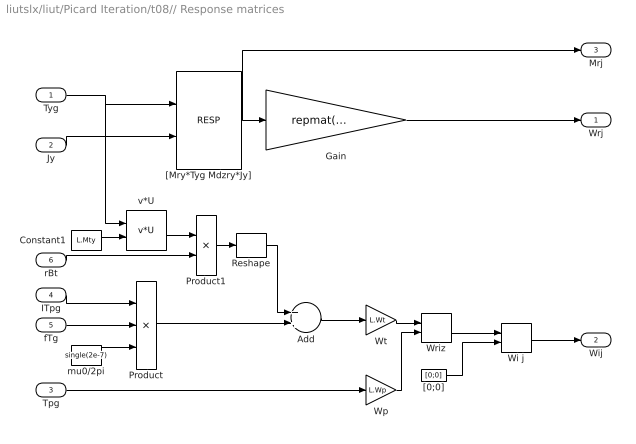
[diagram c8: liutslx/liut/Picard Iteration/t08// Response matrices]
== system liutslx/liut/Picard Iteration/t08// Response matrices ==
  Tyg : Inport
  Jy : Inport  Port=2
  Tpg : Inport  Port=3
  ITpg : Inport  Port=4
  fTg : Inport  Port=5
  rBt : Inport  Port=6
  Add : Sum
  Constant1 : Constant  Value=L.Mty  OutDataTypeStr=single
  Gain : Gain  Gain=repmat(L.Wr,1,L.nj)
  Product : Product  Inputs=3
  Product1 : Product
  Reshape : Reshape  OutputDimensionality=Row vector (2-D)
  Wi j : Concatenate  Mode=Multidimensional array  ConcatenateDimension=2
  Wp : Gain  Gain=L.Wp
  Wriz : Concatenate  Mode=Multidimensional array
  Wt : Gain  Gain=L.Wt
  "[0;0]" : Constant  Value=[0;0]  OutDataTypeStr=single
  "[Mry*Tyg Mdzry*Jy]" : liulib/RESP  A=L.Mry  B=L.Mdzry*L.P.fdz  nr=L.nr  ng=L.ng
  mu0/2pi : Constant  Value=single(2e-7)  OutDataTypeStr=single
  v*U : mkllib/v*U  alpha=1  order=102  transA=112  incx=1  beta=0  incy=1
  Wrj : Outport
  Wij : Outport  Port=2
  Mrj : Outport  Port=3
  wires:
  Reshape/1 -> Add/1
  Constant1/1 -> v*U/2
  Product/1 -> Add/2
  Add/1 -> Wt/1
  Product1/1 -> Reshape/1
  rBt/1 -> Product1/2
  v*U/1 -> Product1/1
  mu0/2pi/1 -> Product/3
  Tyg/1 -> "[Mry*Tyg Mdzry*Jy]"/1, v*U/1
  Jy/1 -> "[Mry*Tyg Mdzry*Jy]"/2
  fTg/1 -> Product/2
  "[Mry*Tyg Mdzry*Jy]"/1 -> Mrj/1, Gain/1
  Wi j/1 -> Wij/1
  "[0;0]"/1 -> Wi j/2
  Wriz/1 -> Wi j/1
  Wt/1 -> Wriz/1
  Wp/1 -> Wriz/2
  Tpg/1 -> Wp/1
  ITpg/1 -> Product/1
  Gain/1 -> Wrj/1

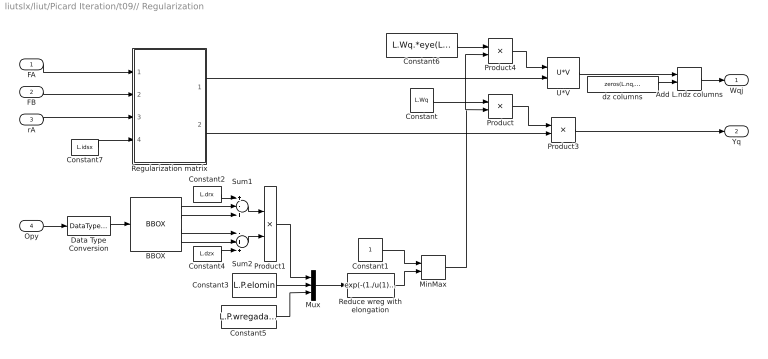
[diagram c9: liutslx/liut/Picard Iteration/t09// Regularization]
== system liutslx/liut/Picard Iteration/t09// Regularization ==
  FA : Inport
  FB : Inport  Port=2
  rA : Inport  Port=3
  Opy : Inport  Port=4
  Add L.ndz columns : Concatenate  Mode=Multidimensional array  ConcatenateDimension=2
  BBOX : liulib/BBOX  z=L.zy  r=L.ry
  Constant : Constant  Value=L.Wq  OutDataTypeStr=single
  Constant1 : Constant  OutDataTypeStr=single
  Constant2 : Constant  Value=L.drx  OutDataTypeStr=single
  Constant3 : Constant  Value=L.P.elomin  OutDataTypeStr=single
  Constant4 : Constant  Value=L.dzx  OutDataTypeStr=single
  Constant5 : Constant  Value=L.P.wregadapt  OutDataTypeStr=single
  Constant6 : Constant  Value=L.Wq.*eye(L.nq)  OutDataTypeStr=single
  Constant7 : Constant  Value=L.idsx  OutDataTypeStr=single
  Data Type Conversion : DataTypeConversion  OutDataTypeStr=boolean
  MinMax : MinMax  Inputs=2
  Mux : Mux  Inputs=3
  Product : Product
  Product1 : Product  Inputs=*/
  Product3 : Product
  Product4 : Product
  Reduce wreg with elongation : Fcn  Expr=exp(-(1./u(1)-u(2))*u(3))
  Regularization matrix : Subsystem  Variant=on  VariantControl=Variant1
  Sum1 : Sum  Inputs=+-+
  Sum2 : Sum  Inputs=-++
  U*V : mkllib/U*V  a=1
  dz columns : Constant  Value=zeros(L.nq,L.ndz)  OutDataTypeStr=single
  Wqj : Outport
  Yq : Outport  Port=2
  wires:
  dz columns/1 -> Add L.ndz columns/2
  Data Type Conversion/1 -> BBOX/1
  Opy/1 -> Data Type Conversion/1
  Constant5/1 -> Mux/3
  Constant3/1 -> Mux/2
  Product1/1 -> Mux/1
  Regularization matrix/1(" Qqg") -> U*V/2
  Product4/1 -> U*V/1
  Regularization matrix/2(" Xq") -> Product3/2
  Product/1 -> Product3/1
  Constant6/1 -> Product4/1
  Mux/1 -> Reduce wreg with elongation/1
  MinMax/1 -> Product/2, Product4/2
  Constant1/1 -> MinMax/1
  Add L.ndz columns/1 -> Wqj/1
  U*V/1 -> Add L.ndz columns/1
  Product3/1 -> Yq/1
  Constant/1 -> Product/1
  Reduce wreg with elongation/1 -> MinMax/2
  BBOX/3 -> Sum2/1
  Constant4/1 -> Sum2/3
  BBOX/2 -> Sum1/3
  BBOX/4 -> Sum2/2
  Sum1/1 -> Product1/1
  Constant2/1 -> Sum1/1
  Sum2/1 -> Product1/2
  BBOX/1 -> Sum1/2
  Constant7/1 -> Regularization matrix/4("ids ")
  rA/1 -> Regularization matrix/3("rA ")
  FB/1 -> Regularization matrix/2("FB ")
  FA/1 -> Regularization matrix/1("FA ")

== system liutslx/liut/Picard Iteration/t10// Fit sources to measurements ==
  Wrj : Inport
  Wij : Inport  Port=2
  Wqj : Inport  Port=3
  Yr : Inport  Port=4
  Yi : Inport  Port=5
  Yq : Inport  Port=6
  Yd : Inport  Port=7
  Ie : Inport  Port=8
  Double precision : Subsystem  VariantControl=liuBSLVMODEvariant2
  Single precision : Subsystem  VariantControl=liuBSLVMODEvariant1
  ag : Outport
  dzg : Outport  Port=2
  Je : Outport  Port=3

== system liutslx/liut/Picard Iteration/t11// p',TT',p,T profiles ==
  ag : Inport
  FA : Inport  Port=2
  FB : Inport  Port=3
  fPg : Inport  Port=4
  fTg : Inport  Port=5
  rBt : Inport  Port=6
  Small diamagnetism approximation : Subsystem
  p',TT',p,hqT profiles : Subsystem  VariantControl=BFCTMODE==1
  PpQ : Outport
  TTpQ : Outport  Port=2
  PQ : Outport  Port=3
  hqTQ : Outport  Port=4
  TQ : Outport  Port=5
  iTQ : Outport  Port=6
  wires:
  fTg/1 -> p',TT',p,hqT profiles/5(fTg)
  FB/1 -> p',TT',p,hqT profiles/3(FB)
  p',TT',p,hqT profiles/3(PQ) -> PQ/1
  p',TT',p,hqT profiles/2(TTpQ) -> TTpQ/1
  p',TT',p,hqT profiles/1(PpQ) -> PpQ/1
  FA/1 -> p',TT',p,hqT profiles/2(FA)
  p',TT',p,hqT profiles/4(hqTQ) -> hqTQ/1, Small diamagnetism approximation/1(hqT)
  rBt/1 -> Small diamagnetism approximation/2(rBt)
  Small diamagnetism approximation/1(T) -> TQ/1  "TQ"
  Small diamagnetism approximation/2(iT) -> iTQ/1  "iTQ"
  ag/1 -> p',TT',p,hqT profiles/1(ag)
  fPg/1 -> p',TT',p,hqT profiles/4(fPg)

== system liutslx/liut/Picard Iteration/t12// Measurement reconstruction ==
  Mrj : Inport
  ag : Inport  Port=2
  dzg : Inport  Port=3
  Ie : Inport  Port=4
  1/fdz : Gain  Gain=1/L.P.fdz
  Add : Sum
  Gain : Gain  Gain=L.Mre  Multiplication=Matrix(K*u) (u vector)
  Selector : Selector  IndexOptions=Index vector (dialog)  Indices=1:L.G.nf  OutputSizes=1
  Selector1 : Selector  IndexOptions=Index vector (dialog)  Indices=L.G.nf + (1:L.G.nm)  OutputSizes=1
  U*v : mkllib/U*v  a=1
  Vector Concatenate : Concatenate
  Bm : Outport
  Ff : Outport  Port=2
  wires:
  1/fdz/1 -> Vector Concatenate/2
  ag/1 -> Vector Concatenate/1
  dzg/1 -> 1/fdz/1
  Vector Concatenate/1 -> U*v/2  "aj"
  Mrj/1 -> U*v/1
  U*v/1 -> Add/1
  Ie/1 -> Gain/1
  Gain/1 -> Add/2
  Add/1 -> Selector1/1, Selector/1
  Selector1/1 -> Bm/1  "Bm"
  Selector/1 -> Ff/1  "Ff"

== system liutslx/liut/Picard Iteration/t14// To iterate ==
  Tyg : Inport
  ag : Inport  Port=2
  Je : Inport  Port=3
  dz : Inport  Port=4
  rst : Inport  Port=5
  Jx : mkllib/U*v  a=1
  Unit Delay : UnitDelay  InitialCondition=1  SampleTime=-1  HasFrameUpgradeWarning=on
  Unit Delay1 : UnitDelay  SampleTime=-1  HasFrameUpgradeWarning=on
  Unit Delay2 : UnitDelay  SampleTime=-1  HasFrameUpgradeWarning=on
  Unit Delay4 : UnitDelay  SampleTime=-1  HasFrameUpgradeWarning=on
  Iy : Outport
  zJy : Outport  Port=2
  zJe : Outport  Port=3
  zdz : Outport  Port=4
  zrst : Outport  Port=5
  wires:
  Unit Delay1/1 -> zdz/1
  Unit Delay4/1 -> zJy/1
  Jx/1 -> Iy/1, Unit Delay4/1  "Iy"
  Tyg/1 -> Jx/1
  dz/1 -> Unit Delay1/1
  ag/1 -> Jx/2
  Unit Delay2/1 -> zJe/1
  Je/1 -> Unit Delay2/1
  Unit Delay/1 -> zrst/1
  rst/1 -> Unit Delay/1

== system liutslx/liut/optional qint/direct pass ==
  LY : Inport
  Fx : Inport  Port=2
  Terminator : Terminator
  LYo : Outport
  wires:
  LY/1 -> LYo/1
  Fx/1 -> Terminator/1

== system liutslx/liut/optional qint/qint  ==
  note: Loop voltage calculation at interpolation points by Finite Differences
  LY : Inport
  Fx : Inport  Port=2
  Add : Sum  Inputs=+-
  Bus Assignment3 : BusAssignment  AssignedSignals=Fn,Brn,Bzn,Brrn,Brzn,Bzrn,Bzzn,Un
  Constant1 : Constant  Value=single(L.P.rn)
  Constant2 : Constant  Value=single(L.P.zn)
  Gain : Gain  Gain=single(1/L.dt)
  Memory : Memory
  QINT : liulib/QINT  rx=L.rx  zx=L.zx  inM=L.inM
  Switch : Switch  Criteria=u2 ~= 0
  LYo : Outport
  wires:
  Bus Assignment3/1 -> LYo/1
  LY/1 -> Bus Assignment3/1
  Constant1/1 -> QINT/2
  Constant2/1 -> QINT/3
  QINT/2 -> Bus Assignment3/3
  QINT/3 -> Bus Assignment3/4
  QINT/4 -> Bus Assignment3/5
  QINT/5 -> Bus Assignment3/6
  QINT/6 -> Bus Assignment3/7
  QINT/7 -> Bus Assignment3/8
  Fx/1 -> QINT/1
  Memory/1 -> Switch/3, Switch/2, Add/2
  QINT/1 -> Memory/1, Add/1, Bus Assignment3/2
  Add/1 -> Gain/1
  Switch/1 -> Bus Assignment3/9
  Gain/1 -> Switch/1

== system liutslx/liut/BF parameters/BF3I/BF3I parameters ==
  Constant : Constant  Value=L.P.bfp.gNg  VectorParams1D=off  OutDataTypeStr=single
  Constant1 : Constant  Value=L.P.bfp.IgNg  VectorParams1D=off  OutDataTypeStr=single
  Constant2 : Constant  Value=L.P.bfp.fPg  OutDataTypeStr=single
  Constant3 : Constant  Value=L.P.bfp.fTg  OutDataTypeStr=single
  gNg : Outport
  IgNg : Outport  Port=2
  fPg : Outport  Port=3
  fTg : Outport  Port=4
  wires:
  Constant1/1 -> IgNg/1
  Constant2/1 -> fPg/1
  Constant3/1 -> fTg/1
  Constant/1 -> gNg/1

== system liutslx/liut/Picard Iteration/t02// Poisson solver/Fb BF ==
  Jy : Inport
  Je : Inport  Port=2
  dz : Inport  Port=3
  ~rst : EnablePort
  Add : Sum  Inputs=+-
  Constant : Constant  Value=0  OutDataTypeStr=single
  Constant1 : Constant  Value=zeros(1,(L.nzy+L.nry)*2+4)  OutDataTypeStr=single
  Divide : Product  Inputs=**
  GSZR BC=0 : Subsystem  TreatAsAtomicUnit=on
  NFDB : liulib/NFDB  nz=L.nzx  nr=L.nrx
  Tbc : mkllib/A*u  A=single(L.Tbc)
  dzMbe : mkllib/A*u  A=single(L.dzMbe)
  =Jy : Outport
  Fb : Outport  Port=2
  =Je : Outport  Port=3
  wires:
  GSZR BC=0/1(Fx) -> NFDB/1
  Constant/1 -> GSZR BC=0/3(dz)
  Constant1/1 -> GSZR BC=0/2(Fb)
  NFDB/1 -> Tbc/1
  Tbc/1 -> Add/1
  Je/1 -> Divide/1, =Je/1
  dz/1 -> Divide/2
  Divide/1 -> dzMbe/1
  Add/1 -> Fb/1
  dzMbe/1 -> Add/2
  Jy/1 -> =Jy/1, GSZR BC=0/1(Iy)

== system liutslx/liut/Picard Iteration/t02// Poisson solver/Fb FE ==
  Yd : Inport
  Ie : Inport  Port=2
  Ip : Inport  Port=3
  sIp : Inport  Port=4
  rst : EnablePort
  FE : liulib/FE  SystemSampleTime=-1
  Mbh* : mkllib/A*u  A=L.Mbh
  Tyh* : mkllib/A*u  A=L.Tyh
  Jy : Outport
  Fb : Outport  Port=2
  Je : Outport  Port=3
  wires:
  FE/1 -> Tyh*/1, Mbh*/1
  sIp/1 -> FE/4
  Ip/1 -> FE/3
  Ie/1 -> FE/2
  FE/2 -> Je/1
  Yd/1 -> FE/1
  Tyh*/1 -> Jy/1
  Mbh*/1 -> Fb/1

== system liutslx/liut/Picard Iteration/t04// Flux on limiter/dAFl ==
  note: % Flux derivative away from axis dAFl = (drFl.*(rA-rl) + dzFl.*(zA-zl));
  drFl : Inport
  rA : Inport  Port=2
  rl : Inport  Port=3
  dzFl : Inport  Port=4
  zA : Inport  Port=5
  zl : Inport  Port=6
  Product : Product
  Product1 : Product
  Sum : Sum  Inputs=|+-
  Sum1 : Sum  Inputs=|+-
  Sum2 : Sum  Inputs=|++
  dAFl : Outport  VectorParamsAs1DForOutWhenUnconnected=on
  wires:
  Sum2/1 -> dAFl/1
  Product/1 -> Sum2/2
  Product1/1 -> Sum2/1
  dzFl/1 -> Product/1
  Sum1/1 -> Product/2
  Sum/1 -> Product1/2
  zl/1 -> Sum1/2
  zA/1 -> Sum1/1
  rl/1 -> Sum/2
  rA/1 -> Sum/1
  drFl/1 -> Product1/1

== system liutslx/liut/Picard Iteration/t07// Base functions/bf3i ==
  Fx : Inport
  Opy : Inport  Port=2
  FA : Inport  Port=3
  FB : Inport  Port=4
  bfp : Inport  Port=5
  err : Inport  Port=6
  BF3I1 : liulib/BF3I1  r=L.ry  ir=L.iry  nz=L.nzy  nr=L.nry
  Demux : Demux  BusSelectionMode=on
  Tyg : Outport
  Tpg : Outport  Port=2
  ITpg : Outport  Port=3
  fPg : Outport  Port=4
  fTg : Outport  Port=5
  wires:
  err/1 -> BF3I1/9
  Demux/4 -> BF3I1/8, fTg/1
  bfp/1 -> Demux/1
  Demux/3 -> fPg/1, BF3I1/7
  Demux/2 -> BF3I1/6
  Demux/1 -> BF3I1/5
  BF3I1/3 -> ITpg/1
  BF3I1/2 -> Tpg/1
  BF3I1/1 -> Tyg/1
  FB/1 -> BF3I1/4
  FA/1 -> BF3I1/3
  Opy/1 -> BF3I1/2
  Fx/1 -> BF3I1/1

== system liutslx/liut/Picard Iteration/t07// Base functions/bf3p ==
  Fx : Inport
  Opy : Inport  Port=2
  FA : Inport  Port=3
  FB : Inport  Port=4
  bfp : Inport  Port=5
  err : Inport  Port=6
  BF3P1 : liulib/BF3P1  ry=L.ry  iry=L.iry  nzy=L.nzy  nry=L.nry
  Constant : Constant  Value=[1 0 0]  VectorParams1D=off  OutDataTypeStr=single
  Constant1 : Constant  Value=[0 1 1]  VectorParams1D=off  OutDataTypeStr=single
  Constant2 : Constant  Value=false
  Terminator : Terminator
  Tyg : Outport
  Tpg : Outport  Port=2
  ITpg : Outport  Port=3
  fPg : Outport  Port=4
  fTg : Outport  Port=5
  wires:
  Constant1/1 -> fTg/1
  Constant/1 -> fPg/1
  bfp/1 -> Terminator/1
  Opy/1 -> BF3P1/2
  Constant2/1 -> BF3P1/5
  BF3P1/2 -> Tpg/1
  BF3P1/3 -> ITpg/1
  BF3P1/1 -> Tyg/1
  Fx/1 -> BF3P1/1
  FA/1 -> BF3P1/3
  FB/1 -> BF3P1/4
  err/1 -> BF3P1/6

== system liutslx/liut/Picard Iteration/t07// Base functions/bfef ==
  Fx : Inport
  Opy : Inport  Port=2
  FA : Inport  Port=3
  FB : Inport  Port=4
  bfp : Inport  Port=5
  err : Inport  Port=6
  BFEF1 : liulib/BFEF1  ry=L.ry  iry=L.iry  nzy=L.nzy  nry=L.nry  nP=L.P.bfp(1)  nT=L.P.bfp(2)
  Constant1 : Constant  Value=L.fTg  OutDataTypeStr=single
  Constant2 : Constant  Value=L.fPg  OutDataTypeStr=single
  Terminator : Terminator
  Tyg : Outport
  Tpg : Outport  Port=2
  ITpg : Outport  Port=3
  fPg : Outport  Port=4
  fTg : Outport  Port=5
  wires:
  bfp/1 -> Terminator/1
  Constant1/1 -> fTg/1
  Constant2/1 -> fPg/1
  BFEF1/1 -> Tyg/1
  BFEF1/2 -> Tpg/1
  BFEF1/3 -> ITpg/1
  err/1 -> BFEF1/5
  FB/1 -> BFEF1/4
  FA/1 -> BFEF1/3
  Opy/1 -> BFEF1/2
  Fx/1 -> BFEF1/1

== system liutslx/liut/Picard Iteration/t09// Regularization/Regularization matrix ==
  "FA " : Inport
  "FB " : Inport  Port=2
  "rA " : Inport  Port=3
  "ids " : Inport  Port=4
  bf3i : Subsystem  VariantControl=liuBFCTMODEvariant2
  bf3p : Subsystem  VariantControl=liuBFCTMODEvariant1
  bfef : Subsystem  VariantControl=liuBFCTMODEvariant3
  " Qqg" : Outport
  " Xq" : Outport  Port=2

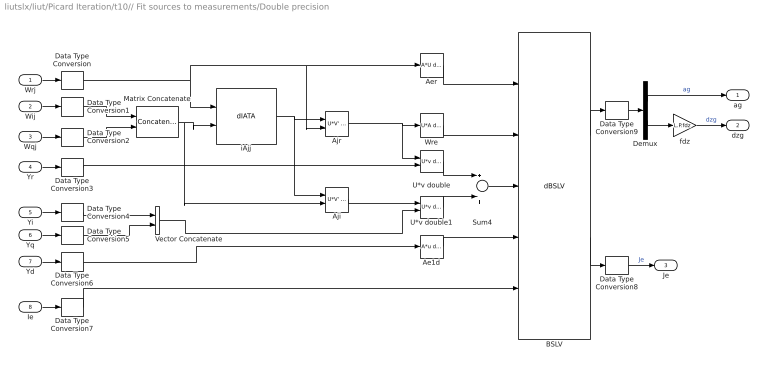
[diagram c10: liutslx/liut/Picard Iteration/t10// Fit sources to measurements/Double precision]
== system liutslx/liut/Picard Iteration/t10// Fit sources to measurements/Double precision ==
  Wrj : Inport
  Wij : Inport  Port=2
  Wqj : Inport  Port=3
  Yr : Inport  Port=4
  Yi : Inport  Port=5
  Yq : Inport  Port=6
  Yd : Inport  Port=7
  Ie : Inport  Port=8
  Ae1d : mkllib/A*u double  A=L.Ae1d
  Aer : mkllib/A*U double  A=L.Aer
  Aji : mkllib/U*V' double  a=1
  Ajr : mkllib/U*V' double  a=1
  BSLV : liulib/dBSLV  niter=L.P.iters
  Data Type Conversion{,1..7} (8 alike) : DataTypeConversion  OutDataTypeStr=double
  Data Type Conversion8 : DataTypeConversion  OutDataTypeStr=single
  Data Type Conversion9 : DataTypeConversion  OutDataTypeStr=single
  Demux : Demux  Outputs=[L.ng L.ndz]
  Matrix Concatenate : Concatenate  Mode=Multidimensional array
  Sum4 : Sum  Inputs=+|+
  U*v double : mkllib/U*v double  a=1
  U*v double1 : mkllib/U*v double  a=1
  Vector Concatenate : Concatenate
  Wre : mkllib/U*A double  A=L.Wre
  fdz : Gain  Gain=L.P.fdz
  iAjj : liulib/dIATA  SFunctionModules=''
  ag : Outport
  dzg : Outport  Port=2
  Je : Outport  Port=3
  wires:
  Vector Concatenate/1 -> U*v double1/2
  Data Type Conversion5/1 -> Vector Concatenate/2
  Data Type Conversion4/1 -> Vector Concatenate/1
  Matrix Concatenate/1 -> iAjj/2, Aji/2
  Data Type Conversion2/1 -> Matrix Concatenate/2
  Data Type Conversion1/1 -> Matrix Concatenate/1
  Wqj/1 -> Data Type Conversion2/1
  Yq/1 -> Data Type Conversion5/1
  Data Type Conversion9/1 -> Demux/1
  Data Type Conversion8/1 -> Je/1  "Je"
  Data Type Conversion7/1 -> BSLV/5
  Data Type Conversion6/1 -> Ae1d/1
  Data Type Conversion3/1 -> U*v double/2
  Data Type Conversion/1 -> Aer/1, Ajr/2, iAjj/1
  fdz/1 -> dzg/1  "dzg"
  iAjj/1 -> Aji/1, Ajr/1
  Sum4/1 -> BSLV/3
  U*v double1/1 -> Sum4/2
  U*v double/1 -> Sum4/1
  Aji/1 -> U*v double1/1
  Yr/1 -> Data Type Conversion3/1
  BSLV/1 -> Data Type Conversion9/1
  Demux/1 -> ag/1  "ag"
  Demux/2 -> fdz/1
  Ie/1 -> Data Type Conversion7/1
  Aer/1 -> BSLV/1
  Wre/1 -> BSLV/2
  Ae1d/1 -> BSLV/4
  BSLV/2 -> Data Type Conversion8/1
  Ajr/1 -> Wre/1, U*v double/1
  Yi/1 -> Data Type Conversion4/1
  Yd/1 -> Data Type Conversion6/1
  Wrj/1 -> Data Type Conversion/1
  Wij/1 -> Data Type Conversion1/1

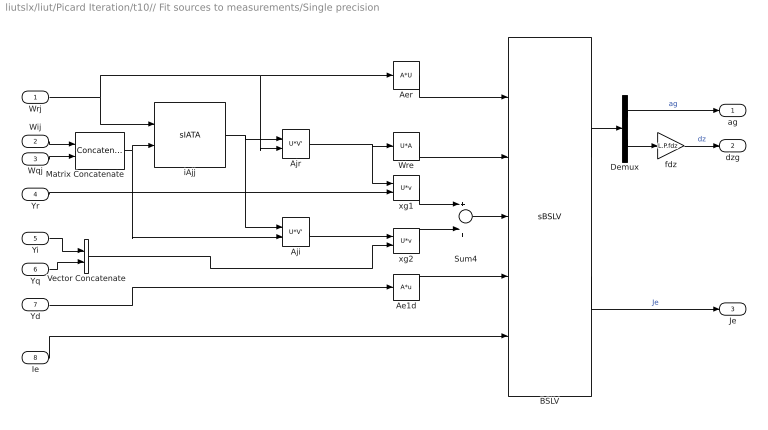
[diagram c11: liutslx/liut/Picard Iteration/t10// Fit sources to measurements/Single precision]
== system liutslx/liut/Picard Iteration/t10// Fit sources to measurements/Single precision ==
  Wrj : Inport
  Wij : Inport  Port=2
  Wqj : Inport  Port=3
  Yr : Inport  Port=4
  Yi : Inport  Port=5
  Yq : Inport  Port=6
  Yd : Inport  Port=7
  Ie : Inport  Port=8
  Ae1d : mkllib/A*u  A=L.Ae1d
  Aer : mkllib/A*U  A=L.Aer
  Aji : mkllib/U*V'  a=1
  Ajr : mkllib/U*V'  a=1
  BSLV : liulib/sBSLV  niter=L.P.iters
  Demux : Demux  Outputs=[L.ng L.ndz]
  Matrix Concatenate : Concatenate  Mode=Multidimensional array
  Sum4 : Sum  Inputs=+|+
  Vector Concatenate : Concatenate
  Wre : mkllib/U*A  A=L.Wre
  fdz : Gain  Gain=L.P.fdz
  iAjj : liulib/sIATA  SFunctionModules=''
  xg1 : mkllib/U*v  a=1
  xg2 : mkllib/U*v  a=1
  ag : Outport
  dzg : Outport  Port=2
  Je : Outport  Port=3
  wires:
  Vector Concatenate/1 -> xg2/2
  Yq/1 -> Vector Concatenate/2
  Yi/1 -> Vector Concatenate/1
  Wqj/1 -> Matrix Concatenate/2
  Wij/1 -> Matrix Concatenate/1
  Matrix Concatenate/1 -> iAjj/2, Aji/2
  fdz/1 -> dzg/1  "dz"
  iAjj/1 -> Ajr/1, Aji/1
  Sum4/1 -> BSLV/3
  xg2/1 -> Sum4/2
  xg1/1 -> Sum4/1
  Aji/1 -> xg2/1
  Yr/1 -> xg1/2
  BSLV/1 -> Demux/1
  Demux/1 -> ag/1  "ag"
  Demux/2 -> fdz/1
  Ie/1 -> BSLV/5
  Aer/1 -> BSLV/1
  Wre/1 -> BSLV/2
  Ae1d/1 -> BSLV/4
  BSLV/2 -> Je/1  "Je"
  Ajr/1 -> Wre/1, xg1/1
  Yd/1 -> Ae1d/1
  Wrj/1 -> Ajr/2, Aer/1, iAjj/1

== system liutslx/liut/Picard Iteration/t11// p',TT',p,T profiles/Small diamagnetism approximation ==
  hqT : Inport
  rBt : Inport  Port=2
  Constant : Constant  OutDataTypeStr=single
  Constant1 : Constant  Value=2  OutDataTypeStr=single
  Sum1 : Sum
  Sum2 : Sum  Inputs=-+
  ahqTg1 : Product
  ahqTg2 : Product
  ahqTg3 : Product
  irBt : Product  Inputs=/*
  T : Outport
  iT : Outport  Port=2
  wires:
  Sum2/1 -> ahqTg3/1
  ahqTg3/1 -> iT/1
  hqT/1 -> ahqTg1/1
  rBt/1 -> Sum1/2, irBt/1
  ahqTg1/1 -> Sum1/1
  Constant/1 -> irBt/2
  Sum1/1 -> T/1, ahqTg2/1
  irBt/1 -> ahqTg1/2, ahqTg3/2, ahqTg2/2
  Constant1/1 -> Sum2/2
  ahqTg2/1 -> Sum2/1

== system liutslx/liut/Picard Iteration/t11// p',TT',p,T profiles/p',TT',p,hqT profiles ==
  ag : Inport
  FA : Inport  Port=2
  FB : Inport  Port=3
  fPg : Inport  Port=4
  fTg : Inport  Port=5
  Base functions on rho grid Coefficients for source terms : Subsystem  Variant=on
  Constant : Constant  Value=L.TQg  VectorParams1D=off  OutDataTypeStr=single
  Constant1 : Constant  Value=L.ITQg  VectorParams1D=off  OutDataTypeStr=single
  smvunv{,1..3} (4 alike) : mkllib/U*v  a=1
  PpQ : Outport
  TTpQ : Outport  Port=2
  PQ : Outport  Port=3
  hqTQ : Outport  Port=4
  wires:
  Constant/1 -> smvunv/1, smvunv1/1
  smvunv1/1 -> TTpQ/1  "TTpQ"
  smvunv3/1 -> hqTQ/1  "hqTQ"
  fTg/1 -> Base functions on rho grid Coefficients for source terms/5(fTg)
  fPg/1 -> Base functions on rho grid Coefficients for source terms/4(fPg)
  Base functions on rho grid Coefficients for source terms/4(ahqTg) -> smvunv3/2
  Base functions on rho grid Coefficients for source terms/3(aPg) -> smvunv2/2
  Base functions on rho grid Coefficients for source terms/2(aTTpg) -> smvunv1/2
  Base functions on rho grid Coefficients for source terms/1(aPpg) -> smvunv/2
  ag/1 -> Base functions on rho grid Coefficients for source terms/1(ag)
  FB/1 -> Base functions on rho grid Coefficients for source terms/3(FB)
  FA/1 -> Base functions on rho grid Coefficients for source terms/2(FA)
  Constant1/1 -> smvunv2/1, smvunv3/1
  smvunv/1 -> PpQ/1  "PpQ"
  smvunv2/1 -> PQ/1  "PQ"

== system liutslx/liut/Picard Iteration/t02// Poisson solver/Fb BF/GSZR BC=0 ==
  note: This subsystem is mecessary to allow treating this as an atomic subsystem. Otherwise we would get improper real-time behaviour
  Iy : Inport
  Fb : Inport  Port=2
  dz : Inport  Port=3
  GSZR : liulib/GSZR  cx=L.cx  cq=L.cq  cr=L.cr  cs=L.cs  ci=L.ci  co=L.co
  Fx : Outport
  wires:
  GSZR/1 -> Fx/1
  Fb/1 -> GSZR/2
  Iy/1 -> GSZR/1
  dz/1 -> GSZR/3

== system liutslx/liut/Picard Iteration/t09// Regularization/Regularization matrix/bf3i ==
  "FA " : Inport
  "FB " : Inport  Port=2
  "rA " : Inport  Port=3
  "ids " : Inport  Port=4
  BF3I6 : liulib/BF3I6  SFunctionModules=''
  Terminator{,1..3} (4 alike) : Terminator
  " Qqg" : Outport
  " Xq" : Outport  Port=2
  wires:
  "ids "/1 -> Terminator3/1
  "rA "/1 -> Terminator2/1
  "FB "/1 -> Terminator1/1
  "FA "/1 -> Terminator/1
  BF3I6/2 -> " Xq"/1
  BF3I6/1 -> " Qqg"/1

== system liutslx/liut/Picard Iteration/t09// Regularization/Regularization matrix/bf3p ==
  "FA " : Inport
  "FB " : Inport  Port=2
  "rA " : Inport  Port=3
  "ids " : Inport  Port=4
  BF3P6 : liulib/BF3P6  SFunctionModules=''
  Divide : Product  Inputs=/
  " Qqg" : Outport
  " Xq" : Outport  Port=2
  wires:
  "rA "/1 -> Divide/1
  BF3P6/1 -> " Qqg"/1
  BF3P6/2 -> " Xq"/1
  "ids "/1 -> BF3P6/4
  Divide/1 -> BF3P6/3
  "FB "/1 -> BF3P6/2
  "FA "/1 -> BF3P6/1

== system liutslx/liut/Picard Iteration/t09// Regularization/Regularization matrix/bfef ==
  "FA " : Inport
  "FB " : Inport  Port=2
  "rA " : Inport  Port=3
  "ids " : Inport  Port=4
  BFEF6 : liulib/BFEF6  nP=L.P.bfp(1)  nT=L.P.bfp(2)  nq=L.nq
  Divide : Product  Inputs=/
  " Qqg" : Outport
  " Xq" : Outport  Port=2
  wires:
  "ids "/1 -> BFEF6/5
  Divide/1 -> BFEF6/4
  "rA "/1 -> BFEF6/3, Divide/1
  "FB "/1 -> BFEF6/2
  "FA "/1 -> BFEF6/1
  BFEF6/2 -> " Xq"/1
  BFEF6/1 -> " Qqg"/1

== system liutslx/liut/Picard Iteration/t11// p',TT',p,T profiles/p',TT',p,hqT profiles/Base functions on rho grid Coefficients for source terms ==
  ag : Inport
  FA : Inport  Port=2
  FB : Inport  Port=3
  fPg : Inport  Port=4
  fTg : Inport  Port=5
  bf3i : Subsystem  VariantControl=liuBFCTMODEvariant2
  bf3p : Subsystem  VariantControl=liuBFCTMODEvariant1
  bfef : Subsystem  VariantControl=liuBFCTMODEvariant3
  aPpg : Outport
  aTTpg : Outport  Port=2
  aPg : Outport  Port=3
  ahqTg : Outport  Port=4

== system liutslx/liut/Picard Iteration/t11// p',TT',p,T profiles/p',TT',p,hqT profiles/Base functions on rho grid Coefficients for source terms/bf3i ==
  ag : Inport
  FA : Inport  Port=2
  FB : Inport  Port=3
  fPg : Inport  Port=4
  fTg : Inport  Port=5
  BF3I3 : liulib/BF3I3  idsx=L.idsx
  aPpg : Outport
  aTTpg : Outport  Port=2
  aPg : Outport  Port=3
  ahqTg : Outport  Port=4
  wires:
  BF3I3/4 -> ahqTg/1
  BF3I3/3 -> aPg/1
  BF3I3/2 -> aTTpg/1
  BF3I3/1 -> aPpg/1
  FB/1 -> BF3I3/3
  FA/1 -> BF3I3/2
  ag/1 -> BF3I3/1
  fTg/1 -> BF3I3/5
  fPg/1 -> BF3I3/4
